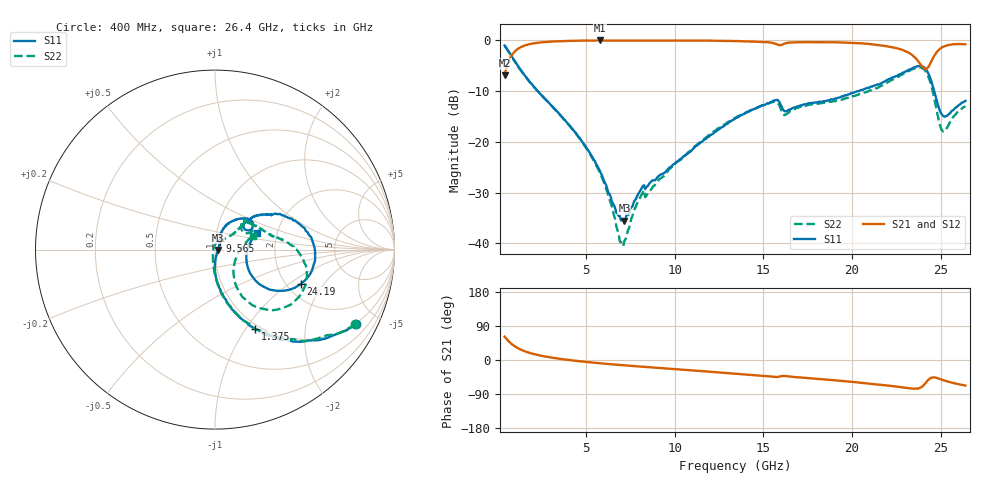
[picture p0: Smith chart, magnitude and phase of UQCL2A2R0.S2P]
! AVX Corporation
! Date:  10/27/06
! Part No:  UQCL2A2R0
! Description:  Ultra Low ESR Microwave capacitors
! Mounting Orientation:  Horizontal
# GHZ S DB R 50
! Freq  |S11|  S11 Ph  |S21|  S21 Ph  |S12|  S12 Ph  |S22|  S22 Ph
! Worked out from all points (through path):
!   401 points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, 400 MHz to 26.4 GHz, reference 50 ohm
!   highest |S21| = -0.02 dB at 5.795 GHz (marker M1); lowest = -6.8 dB at 400 MHz (marker M2)
!   group delay of S21, straight-line fit = 9.98 ps
!   lowest |S11| = -35.5 dB at 7.16 GHz (marker M3), VSWR 1.03, Z = 51.7 - j0.156 ohm
!   |S11| at or under -10 dB: 2.279 GHz to 20.33 GHz (18.05 GHz wide, 160 % of centre); 24.64 GHz to end of sweep
!   |S22| runs from -40.5 to -1.1 dB; largest |S21 - S12| = 0.015
!   S11 on the Smith chart (normalised r, x): 400 MHz: 0.95, -3.79; 1.375 GHz: 0.95, -1.10; 9.565 GHz: 1.05, +0.10; 24.19 GHz: 2.37, -1.24; 26.4 GHz: 1.58, +0.32
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0.4  -1.02 -28.0  -6.85 61.6  -6.90 61.5  -1.07 -28.0
0.79  -3.05 -46.9  -2.98 42.5  -3.04 42.1  -3.16 -47.2
1.375  -6.14 -63.2  -1.24 26.1  -1.27 26.1  -6.22 -63.5
2.545  -11.00 -78.1  -0.38 10.5  -0.39 10.7  -11.06 -79.3
4.755  -19.87 -90.5  -0.05 -3.8  -0.05 -3.9  -19.91 -93.6
5.795  -25.89 -86.1  -0.02 -8.7  -0.04 -8.7  -26.21 -104.2
6.315  -30.24 -74.2  -0.02 -10.8  -0.04 -10.5  -31.29 -113.2
6.9  -34.59 -32.3  -0.02 -13.1  -0.01 -13.0  -39.60 -157.4
7.16  -35.50 -5.2  -0.03 -14.1  -0.01 -14.0  -39.47 153.8
8.135  -29.09 43.0  -0.03 -17.6  -0.01 -17.7  -30.38 90.4
9.11  -26.66 54.9  -0.04 -21.0  -0.02 -21.1  -27.40 72.6
9.565  -25.58 60.9  -0.05 -22.5  -0.03 -22.6  -25.98 66.4
13.4  -15.46 61.7  -0.15 -36.0  -0.12 -36.1  -15.28 41.6
15.675  -11.81 39.5  -0.66 -44.8  -0.67 -45.3  -12.10 33.0
16.195  -13.94 34.0  -0.64 -42.1  -0.66 -42.6  -14.72 35.0
17.755  -12.29 41.0  -0.36 -48.8  -0.46 -49.2  -12.61 41.4
22.11  -7.58 27.7  -1.25 -68.1  -1.30 -67.8  -8.08 6.6
23.605  -5.21 3.3  -3.57 -75.8  -3.60 -75.4  -5.45 -17.0
24.19  -5.77 -21.9  -5.63 -58.9  -5.64 -58.5  -6.30 -43.5
24.645  -10.06 -38.0  -3.02 -46.0  -3.05 -45.8  -11.42 -60.2
25.1  -14.74 -17.1  -1.35 -52.4  -1.38 -52.0  -17.85 -28.7
26.4  -11.91 21.6  -0.78 -67.3  -0.78 -66.9  -13.00 20.1
